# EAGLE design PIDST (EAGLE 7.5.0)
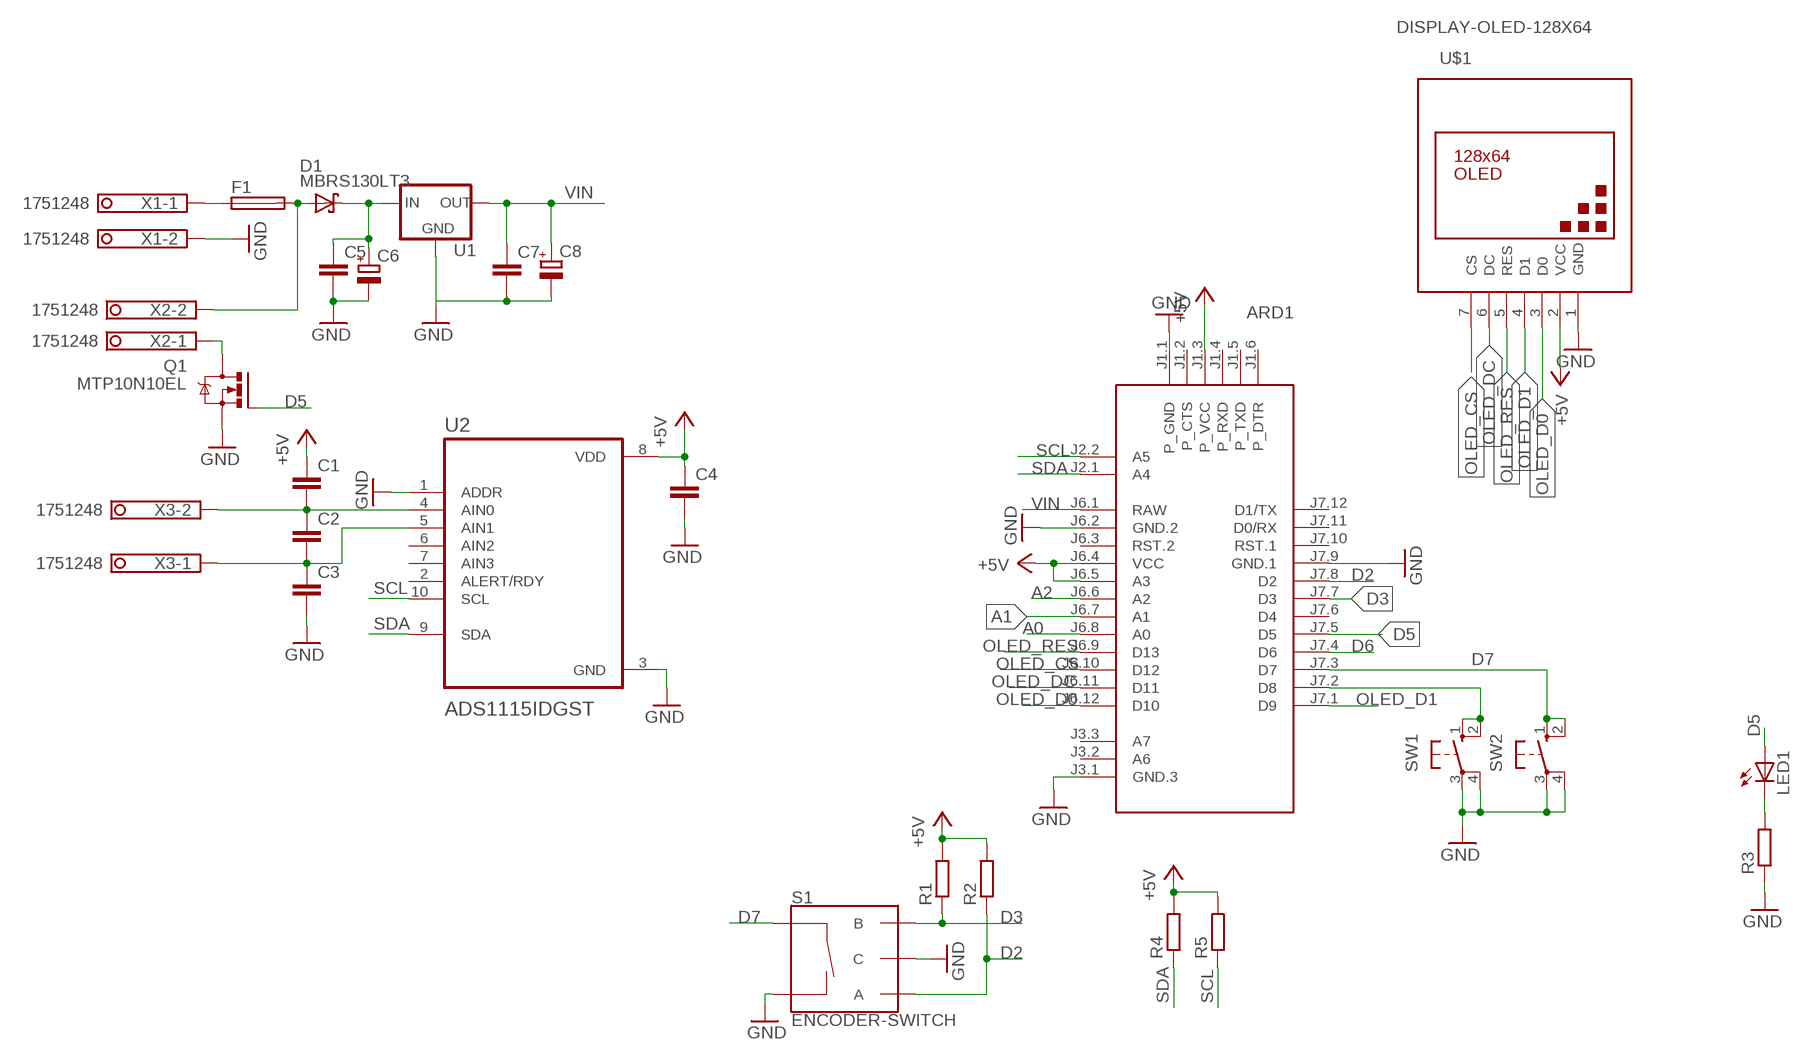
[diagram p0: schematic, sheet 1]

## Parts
ARD1  ARDUINO-PRO-MINI-3.3V  [ARDUINO-PRO-MINI]
C1  C-EUC1206  [C1206]
C2  C-EUC1206  [C1206]
C3  C-EUC1206  [C1206]
C4  C-EUC1206  [C1206]
C5  C-EUC1206  [C1206]
C6  CPOL-EUSMCB  [SMC_B]
C7  C-EUC1206  [C1206]
C8  CPOL-EUSMCB  [SMC_B]
D1  MBRS130LT3  [SMB]
F1  SH22,5  [SH22,5]
LED1  LED5MM  [LED5MM]
Q1  MTP10N10EL  IRLZ44Z  [TO220BH]
R1  R-EU_R1206  [R1206]
R2  R-EU_R1206  [R1206]
R3  R-EU_R1206  [R1206]
R4  R-EU_R1206  [R1206]
R5  R-EU_R1206  [R1206]
S1  ENCODER-SWITCH  [ROTARY_ENC_PLAIN]
SW1  10-XX  [B3F-10XX]
SW2  10-XX  [B3F-10XX]
U1  78LXX  [78LXX]
U2  ADS1115IDGST  [SOP50P490X110-10N]
U$1  DISPLAY-OLED-128X64  [DISPLAY-OLED-128X64]
X1  1751248  [1751248]
X2  1751248  [1751248]
X3  1751248  [1751248]

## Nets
+5V: ARD1.J1.3(P_VCC) ARD1.J6.4(VCC) ARD1.J6.5(A3) C1.1 C4.1 R1.2 R2.2 R4.2 R5.2 U2.8(VDD) U$1.2(VCC)
A0: ARD1.J6.8(A0)
A1: ARD1.J6.7(A1)
A2: ARD1.J6.6(A2)
D2: ARD1.J7.8(D2) R2.1 S1.A
D3: ARD1.J7.7(D3) R1.1 S1.B
D5: ARD1.J7.5(D5) LED1.A Q1.G
D6: ARD1.J7.4(D6)
D7: ARD1.J7.3(D7) S1.SW+ SW2.1(S) SW2.2(S1)
GND: ARD1.J1.1(P_GND) ARD1.J3.1(GND.3) ARD1.J6.2(GND.2) ARD1.J7.9(GND.1) C3.2 C4.2 C5.2 C6.- C7.2 C8.- Q1.S R3.1 S1.C S1.SW- SW1.3(P) SW1.4(P1) SW2.3(P) SW2.4(P1) U1.GND U2.1(ADDR) U2.3(GND) U$1.1(GND) X1.2
N$1: C1.2 C2.1 U2.4(AIN0) X3.2
N$2: C2.2 C3.1 U2.5(AIN1) X3.1
N$3: Q1.D X2.1
N$4: F1.1 X1.1
N$5: D1.A F1.2 X2.2
N$6: C5.1 C6.+ D1.C U1.IN
N$7: LED1.K(C) R3.2
N$8: ARD1.J7.2(D8) SW1.1(S) SW1.2(S1)
OLED_CS: ARD1.J6.10(D12) U$1.7(CS)
OLED_D0: ARD1.J6.12(D10) U$1.3(D0)
OLED_D1: ARD1.J7.1(D9) U$1.4(D1)
OLED_DC: ARD1.J6.11(D11) U$1.6(DC)
OLED_RES: ARD1.J6.9(D13) U$1.5(RES)
SCL: ARD1.J2.2(A5) R5.1 U2.10(SCL)
SDA: ARD1.J2.1(A4) R4.1 U2.9(SDA)
VIN: ARD1.J6.1(RAW) C7.1 C8.+ U1.OUT
Unconnected: ARD1.J1.2(P_CTS) ARD1.J1.4(P_RXD) ARD1.J1.5(P_TXD) ARD1.J1.6(P_DTR) ARD1.J3.2(A6) ARD1.J3.3(A7) ARD1.J6.3(RST.2) ARD1.J7.6(D4) ARD1.J7.10(RST.1) ARD1.J7.11(D0/RX) ARD1.J7.12(D1/TX) U2.2(ALERT/RDY) U2.6(AIN2) U2.7(AIN3)

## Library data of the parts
ARD1 = diy-modules:ARDUINO-PRO-MINI-*: Arduino Pro Mini and compatible devices More details available here: https://www.arduino.cc/en/Main/ArduinoBoardProMini Click here to find device on ebay.com
C1-C5 C7 = rcl:C-EU: CAPACITOR, European symbol
C6 C8 = rcl:CPOL-EU: POLARIZED CAPACITOR, European symbol
D1 = diode:MBRS130LT3: Schottky Power Rectifier
F1 = fuse:SH22,5: FUSE HOLDER; MF: SCHURTER; MPN: 0031.8201; OC_FARNELL: 1162740; OC_NEWARK: 96F8317
LED1 = led:LED: LED
Q1 = transistor-power:IRLZ44Z: N-Channel HEXFET® Power MOSFET Logic Level AUTOMOTIVE MOSFET Source: http://www.irf.com/product-info/datasheets/data/irlz44zpbf.pdf
R1-R5 = rcl:R-EU_: RESISTOR, European symbol
S1 = SparkFun-Switches:ENCODER-SWITCH: Rotary Encoder w/ Select Switch Encoders rotate similarly to potentiometers, but they’re different from potentiometers in that an encoder has full rotation without limits. They output gray code so that you can tell how much and in which direction the encoder has been turned. This encoder includes a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; SF_SKU: COM-09117
SW1 SW2 = switch-omron:10-XX: OMRON SWITCH; MPN: B3F-1000; OC_FARNELL: 176432; OC_NEWARK: 36M3542
U1 = v-reg:78LXX: VOLTAGE REGULATOR
U2 = ADS1115IDGST:ADS1115IDGST: Check availability; AVAILABILITY: In Stock; CHECK_PRICES: https://www.snapeda.com/parts/ADS1115IDGST/Texas+Instruments/view-part/?ref=eda; DESCRIPTION: 16-bit, 860-SPS, 4-channel, delta-sigma ADC with PGA, oscillator, VREF, comparator and I2C; MF: Texas Instruments; MP: ADS1115IDGST; PACKAGE: VSSOP-10 Texas Instruments; PRICE: None; SNAPEDA_LINK: https://www.snapeda.com/parts/ADS1115IDGST/Texas+Instruments/view-part/?ref=snap
U$1 = diy-modules:DISPLAY-OLED-128X64: 128x64 Dot Matrix OLED Module based on SSD1306 chip Variant with SPI interface More details available here: http://www.instructables.com/id/How-to-use-OLED-display-arduino-module/ SSD1306 datasheet: https://cdn-shop.adafruit.com/datasheets/SSD1306.pdf Click here to find device on ebay.com Note: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
X1-X3 = con-phoenix-350:1751248: MKDS 1/ 2-3,5 Printklemme; OC_FARNELL: unknown; OC_NEWARK: unknown

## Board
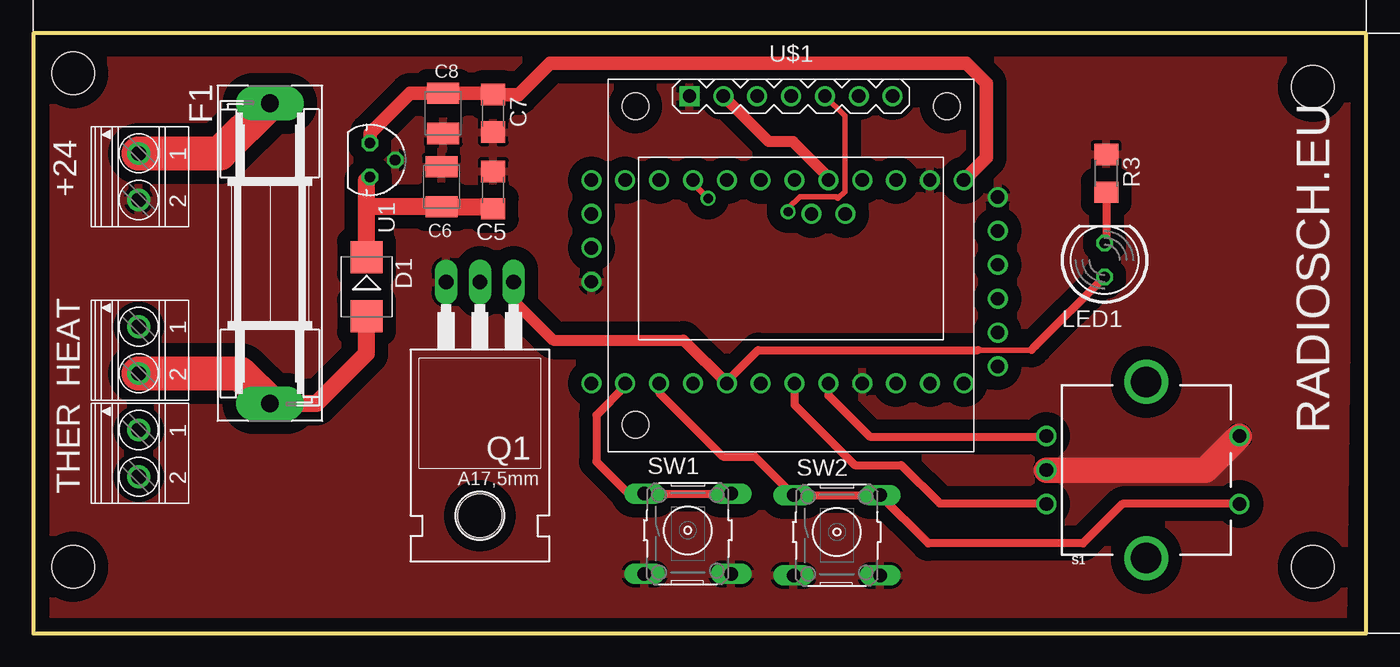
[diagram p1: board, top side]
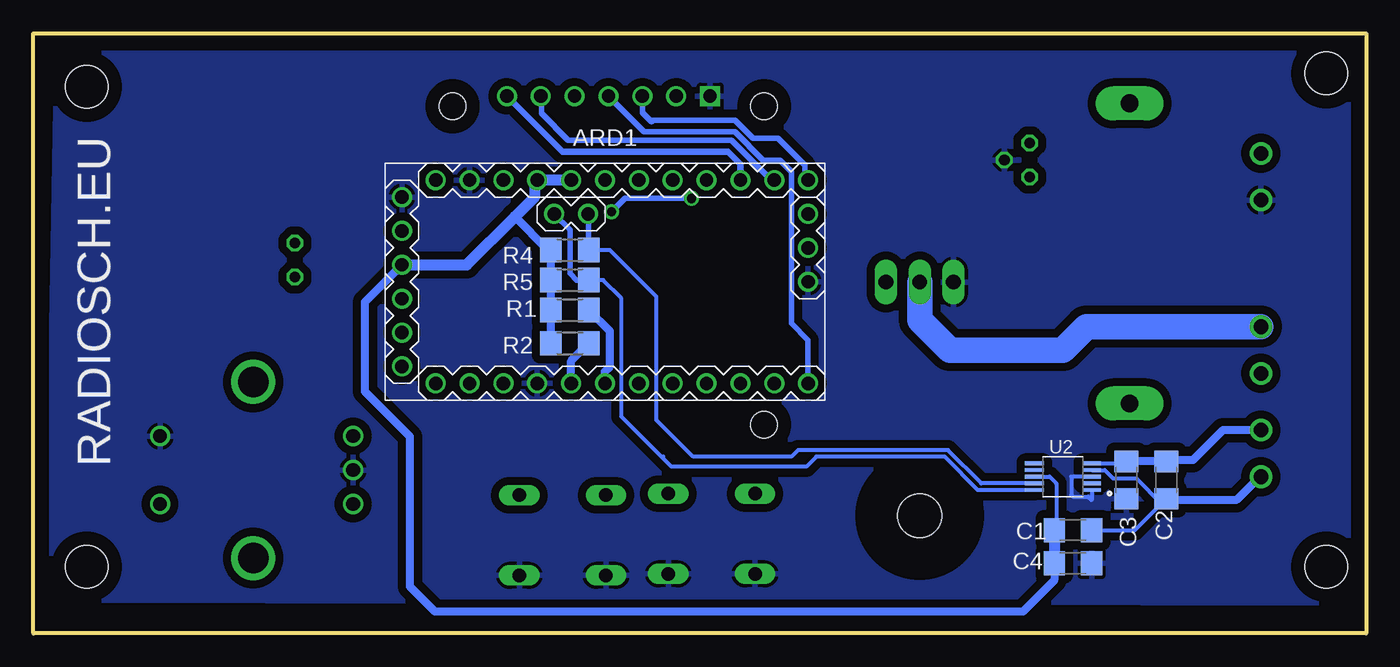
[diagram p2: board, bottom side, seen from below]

Size 100 x 45 mm. Coordinates in mm from the lower left corner, seen from the top.
Outline: 0,0 100,0 100,45 0,45 0,0
Copper layers (1*16): Top 0.035mm / dielectric 1.5mm / Bottom 0.035mm
Design rules "default *": minimum track width 10mil, minimum drill 24mil, track to track 6mil, track to pad 8mil, pad to pad 8mil, via to via 8mil, smd to smd 8mil, copper to edge 40mil, drill to drill 8mil, minimum pad ring 8mil, minimum via ring 8mil, stop-mask expansion 4mil, vias tented up to drill 0mil, thermal gap 10mil
Holes 3.2 mm at 3,42 3,5 96,5 96,41

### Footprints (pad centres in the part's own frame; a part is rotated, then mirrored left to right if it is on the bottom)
ARDUINO-PRO-MINI = drill 1: J1.1 -15.24,6.35; J1.2 -15.24,3.81; J1.3 -15.24,1.27; J1.4 -15.24,-1.27; J1.5 -15.24,-3.81; J1.6 -15.24,-6.35; J2.1 -1.27,5.08; J2.2 -3.81,5.08; J3.1 15.24,0; J3.2 15.24,2.54; J3.3 15.24,5.08; J6.1 -12.7,7.62; J6.2 -10.16,7.62; J6.3 -7.62,7.62; J6.4 -5.08,7.62; J6.5 -2.54,7.62; J6.6 0,7.62; J6.7 2.54,7.62; J6.8 5.08,7.62; J6.9 7.62,7.62; J6.10 10.16,7.62; J6.11 12.7,7.62; J6.12 15.24,7.62; J7.1 15.24,-7.62; J7.2 12.7,-7.62; J7.3 10.16,-7.62; J7.4 7.62,-7.62; J7.5 5.08,-7.62; J7.6 2.54,-7.62; J7.7 0,-7.62; J7.8 -2.54,-7.62; J7.9 -5.08,-7.62; J7.10 -7.62,-7.62; J7.11 -10.16,-7.62; J7.12 -12.7,-7.62
C1206 = smd 1.6 x 1.8: 1 -1.4,0; 2 1.4,0
SMC_B = smd 1.6 x 2.4: + -1.5,0; - 1.5,0
SMB = smd 2.4 x 2.4: A 2.2,0; C -2.2,0
SH22,5 = drill 1.321 pad 2.54 long: 1 -11.252,0; 2 11.252,0
LED5MM = drill 0.813 octagon: A -1.27,0; K 1.27,0
TO220BH = drill 1.118 long: D 0,-6.35; G -2.54,-6.35; S 2.54,-6.35 | hole 3.302: 0,11.176
R1206 = smd 1.6 x 1.803: 1 -1.422,0; 2 1.422,0
ROTARY_ENC_PLAIN = drill 1.016: A 7.493,-2.54; B 7.493,2.54; C 7.493,0; SW+ -6.985,2.54; SW- -6.985,-2.54 | drill 2.286: P$3 0,6.604; P$4 0,-6.604
B3F-10XX = drill 1.016 long: 1 -3.251,2.761; 2 3.251,2.761; 3 -3.251,-3.261; 4 3.251,-3.261
78LXX = drill 0.813 octagon: GND 0,1.905; IN 1.27,0; OUT -1.27,0
SOP50P490X110-10N = smd 1.47 x 0.28: 1 -2.15,1; 2 -2.15,0.5; 3 -2.15,0; 4 -2.15,-0.5; 5 -2.15,-1; 6 2.15,-1; 7 2.15,-0.5; 8 2.15,0; 9 2.15,0.5; 10 2.15,1
DISPLAY-OLED-128X64 = drill 1 square: 1 -7.62,12.7 | drill 1: 2 -5.08,12.7; 3 -2.54,12.7; 4 0,12.7; 5 2.54,12.7; 6 5.08,12.7; 7 7.62,12.7 | hole 2: -11.684,11.938; 11.684,11.938; -11.684,-11.938
1751248 = drill 1.1 pad 1.7: 1 -1.75,-0.1; 2 1.75,-0.1

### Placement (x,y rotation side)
ARD1  57.11,26.37 0 bottom
C1  22,7.75 0 bottom
C2  15,11.5 90 bottom
C3  18,11.5 270 bottom
C4  22,5.25 0 bottom
C5  34.5,33.25 90 top
C6  30.62,33.5 90 top
C7  34.5,39 270 top
C8  30.75,39 270 top
D1  25,26 270 top
F1  17.75,28.5 270 top
LED1  80.38,28 90 top
Q1  33.5,20 180 top
R1  59.75,24.25 180 bottom
R2  59.75,21.75 180 bottom
R3  80.5,34.5 270 top
R4  59.75,28.75 180 bottom
R5  59.75,26.5 180 bottom
S1  83.5,12.25 180 top
SW1  49.1,7.72 0 top
SW2  60.28,7.6 0 top
U1  25.25,35.5 270 top
U2  22.75,11.75 180 bottom
U$1  56.85,27.59 0 top
X1  8,34.25 270 top
X2  8,21.25 270 top
X3  8,13.5 270 top

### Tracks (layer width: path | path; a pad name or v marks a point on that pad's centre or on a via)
+5V
  Top 0.813: ARD1.J6.5 59.65,34.23 57,36.88 55.19,36.88 U$1.2
  Bottom 0.305: U2.8 23.75,11.75 23.25,11.25 23.25,7.9 C1.1
  Bottom 0.61: C4.1 23.4,3.98 25.75,1.62 69.88,1.62 71.75,3.5 71.75,14.75 75.12,18.12 75.12,24.86 ARD1.J1.3 | R2.2 R1.2 R5.2 R4.2 61.38,28.75 63.88,31.25
  Bottom 0.813: ARD1.J6.5 ARD1.J6.4 62.38,33.8 62.38,32.75 63.88,31.25 67.48,27.64 ARD1.J1.3 | C1.1 C4.1
D2
  Top 0.61: ARD1.J7.8 59.65,17.85 62.75,14.75 75.97,14.75 S1.A
  Bottom 0.61: ARD1.J7.8 59.65,20.43 R2.1
D3
  Top 0.61: ARD1.J7.7 57.11,17.14 61.62,12.62 65.12,12.62 68,9.75 75.97,9.75 S1.B
  Bottom 0.61: ARD1.J7.7 57.11,19.64 56.75,20 56.75,22.67 R1.1
D5
  Top 0.406: 70.88,21.25 74.89,21.25
  Top 0.61: ARD1.J7.5 52.03,18.91 54.38,21.25 70.88,21.25 | 74.89,21.25 75.2,21.55 LED1.A
  Top 0.813: Q1.G 36.04,24.96 39,22 48.78,22 ARD1.J7.5
D7
  Top 0.61: ARD1.J7.3 46.95,18.05 51.75,13.25 54.14,13.25 SW2.1 SW2.2 67.15,6.75 78.75,6.75 81.71,9.71 S1.SW+
GND
  Top 1.93: S1.C 87.94,12.25 S1.SW-
  Bottom 0.305: U2.1 20.6,10.03 20.62,10 20.88,10.25 22,10.25 22.12,10.38 22.12,11.75 U2.3
  pour Top (isolate 1.016): 1,43 98.75,43 98.25,0.5 1.5,0.5
  pour Bottom (isolate 0.61): 1.25,43.5 98.25,43.5 99,2.5 0.5,2.25
N$1
  Bottom 0.305: C1.2 17.35,7.75 15.36,9.74 | 15.36,9.74 C2.1 | U2.4 19.62,12.25 19,11.62 17.25,11.62 15.36,9.74
  Bottom 0.61: X3.2 8,11.75 9.75,10 14.9,10 C2.1
N$2
  Bottom 0.305: U2.5 18.15,12.75 C3.1
  Bottom 0.61: C3.1 C2.2 14.9,13 13,13 10.75,15.25 X3.1
N$3
  Bottom 1.93: X2.1 21,23 22.75,21.25 31.25,21.25 33.5,23.5 Q1.D
N$4
  Top 2.54: X1.1 14,36 F1.1
N$5
  Top 1.27: F1.2 21.25,17.25 25,21 D1.A
  Top 2.54: F1.2 15.5,19.5 X2.2
N$6
  Top 1.27: D1.C 25,32.25 | 25,32.25 25,33.98 U1.IN | 25,32.25 25.25,32 C6.+ 34.35,32 C5.1
N$7
  Top 0.61: R3.2 80.5,29.39 LED1.K
N$8
  Top 0.61: ARD1.J7.2 44.41,18.54 42.25,16.38 42.25,12.88 44.75,10.38 45.74,10.38 SW1.1 SW1.2
OLED_CS
  Bottom 0.5: ARD1.J6.10 46.95,35.2 47.88,36.12 60.3,36.12 U$1.7
OLED_D0
  Bottom 0.406: U$1.3 54.31,39.06 53.62,38.38 53.5,38.5 47.38,38.5 46,37.12 44.12,37.12 42.12,35.12 42.12,34.25 ARD1.J6.12
OLED_D1
  Bottom 0.406: ARD1.J7.1 41.87,21.99 43.12,23.25 43.12,34.62 44,35.5 45.25,35.5 47.38,37.62 54.19,37.62 U$1.4
OLED_DC
  Bottom 0.406: ARD1.J6.11 44.62,33.99 47.62,37 59.88,37 61.88,39 61.88,40.23 U$1.6
OLED_RES  (via drill 0.7)
  Top 0.406: U$1.5 60.88,38.8 60.88,33.12 60.38,32.62 60.25,32.75 57.5,32.75 56.62,31.88 v56.62,31.62
  Top 0.5: ARD1.J6.9 49.49,33.76 v50.62,32.62
  Bottom 0.406: v50.62,32.62 55.62,32.62 v56.62,31.62
SCL
  Bottom 0.305: U2.10 29.12,10.75 31.62,13.25 41.25,13.25 42,12.5 52.12,12.5 52.81,13.19 | 52.5,12.88 52.81,13.19 | 52.81,13.19 52.88,13.25 55.88,16.25 55.88,25.12 57.25,26.5 R5.1 | 52.75,13.25 52.81,13.19
  Bottom 0.406: R5.1 59.25,26.5 59.75,27 59.75,30.28 ARD1.J2.2
SDA
  Bottom 0.305: U2.9 28.88,11.25 31.38,13.75 42.62,13.75 43.12,13.25 50.5,13.25 53.25,16 53.25,25.25 56.75,28.75 R4.1
  Bottom 0.406: R4.1 58.33,31.4 ARD1.J2.1
VIN
  Top 1.016: U1.OUT 25.25,37.5 28.25,40.5 C8.+ 34.4,40.5 C7.1 36.4,40.4 38.75,42.75 70,42.75 71.5,41.25 71.5,35.68 ARD1.J6.1

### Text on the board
tPlace: +24 | HEAT | RADIOSCH.EU | THER
bPlace: RADIOSCH.EU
